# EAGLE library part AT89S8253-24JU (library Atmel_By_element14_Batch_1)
Microcontroller
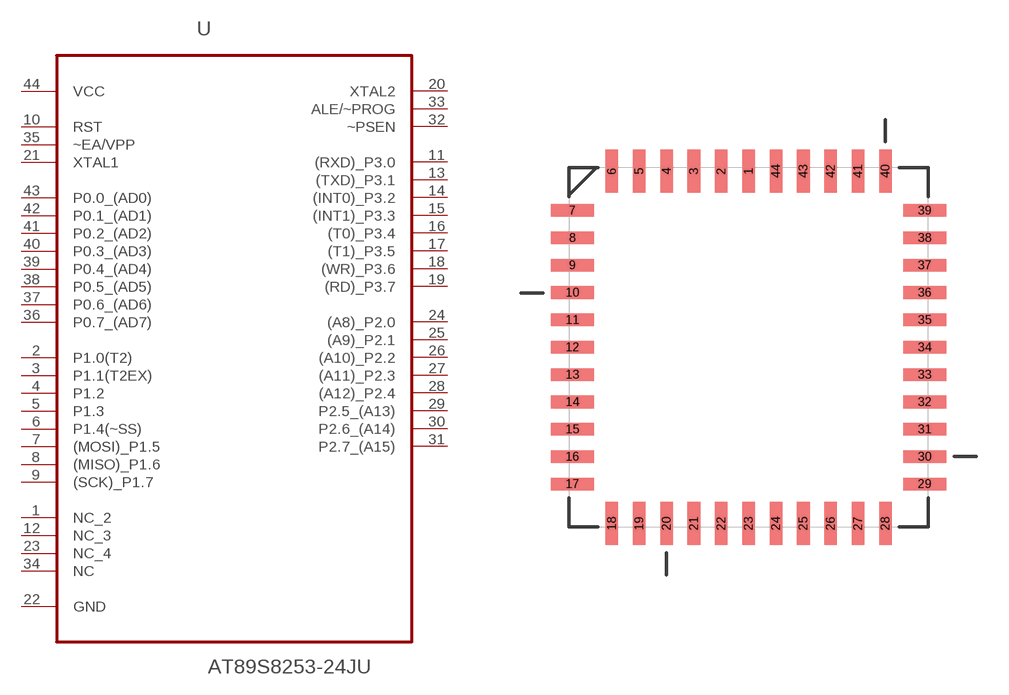
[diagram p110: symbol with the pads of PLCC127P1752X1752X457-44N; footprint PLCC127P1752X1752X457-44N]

Designator prefix U

## AT89S8253-24JU (DESCRIPTION: Microcontroller; MPN: AT89S8253-24JU; OC_FARNELL: 1095745; OC_NEWARK: 96K6581; PACKAGE: PLCC-44; SUPPLIER: ATMEL)  [PLCC127P1752X1752X457-44N]
1  NC_2  nc
2  P1.0(T2)
3  P1.1(T2EX)
4  P1.2
5  P1.3
6  P1.4(~SS)
7  (MOSI)_P1.5
8  (MISO)_P1.6
9  (SCK)_P1.7
10  RST  in
11  (RXD)_P3.0
12  NC_3  nc
13  (TXD)_P3.1
14  (INT0)_P3.2
15  (INT1)_P3.3
16  (T0)_P3.4
17  (T1)_P3.5
18  (WR)_P3.6
19  (RD)_P3.7
20  XTAL2  out
21  XTAL1  in
22  GND  pas
23  NC_4  nc
24  (A8)_P2.0
25  (A9)_P2.1
26  (A10)_P2.2
27  (A11)_P2.3
28  (A12)_P2.4
29  P2.5_(A13)
30  P2.6_(A14)
31  P2.7_(A15)
32  ~PSEN  out
33  ALE/~PROG  out
34  NC  nc
35  ~EA/VPP  in
36  P0.7_(AD7)
37  P0.6_(AD6)
38  P0.5_(AD5)
39  P0.4_(AD4)
40  P0.3_(AD3)
41  P0.2_(AD2)
42  P0.1_(AD1)
43  P0.0_(AD0)
44  VCC  pwr

## Footprint PLCC127P1752X1752X457-44N (pad centres in mm)
smd 0.584 x 2.007: 1 0,8.179; 2 -1.27,8.179; 3 -2.54,8.179; 4 -3.81,8.179; 5 -5.08,8.179; 6 -6.35,8.179; 18 -6.35,-8.179; 19 -5.08,-8.179; 20 -3.81,-8.179; 21 -2.54,-8.179; 22 -1.27,-8.179; 23 0,-8.179; 24 1.27,-8.179; 25 2.54,-8.179; 26 3.81,-8.179; 27 5.08,-8.179; 28 6.35,-8.179; 40 6.35,8.179; 41 5.08,8.179; 42 3.81,8.179; 43 2.54,8.179; 44 1.27,8.179
smd 2.007 x 0.584: 7 -8.179,6.35; 8 -8.179,5.08; 9 -8.179,3.81; 10 -8.179,2.54; 11 -8.179,1.27; 12 -8.179,0; 13 -8.179,-1.27; 14 -8.179,-2.54; 15 -8.179,-3.81; 16 -8.179,-5.08; 17 -8.179,-6.35; 29 8.179,-6.35; 30 8.179,-5.08; 31 8.179,-3.81; 32 8.179,-2.54; 33 8.179,-1.27; 34 8.179,0; 35 8.179,1.27; 36 8.179,2.54; 37 8.179,3.81; 38 8.179,5.08; 39 8.179,6.35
